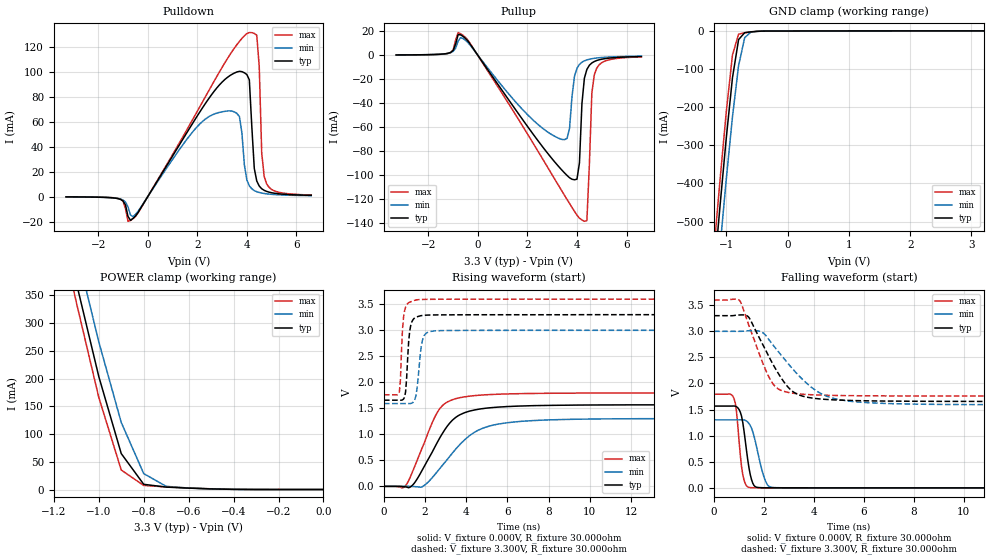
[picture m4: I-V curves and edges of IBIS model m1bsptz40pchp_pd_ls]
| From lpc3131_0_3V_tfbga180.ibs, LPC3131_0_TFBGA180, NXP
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| |   Rev 0.20 IBIS Model Design Automation Generation   |
| |   N O N - S I L I C O N   C O R R E L A T E D   |
| |   This IBIS [Model] is pre-Beta tactical support   |
| |  Note: this IBIS [Model] contains clamp curves generated   |
| |   through simulation which should not be relied upon   |
| Date/Time   : 2010 Jan 25 (Mon) 11:58:19
| Pccmos090 jliolib_p50 2.0
|   0.9 um 3.3V pad library
|   seven level metal
|   dual oxide
|   dual threshold voltage
|   nominal line mixed supply
|   parasitic extracted netlists
| Process block a10
| mem1bsptz40pchp
|   Bidirectional Pad 3.3
|   3state Output
|   Plain Input
|   CMOS
|   Programmable between
|   - (p1=0, p2=1) plain input
|   - (p1=0, p2=0) with Pull Up
|   - (p1=1, p2=1) with Pull Down
|   - (p1=1, p2=0) with Repeater
| Pull Down Mode low speed(esh=1, p1=1, p2=1)
[Model]   m1bsptz40pchp_pd_ls | of mem1bsptz40pchp
Model_type   I/O
Polarity   Non-Inverting
Enable   Active-Low
|  Reciever Thresholds
Vinl   = 0.99V
Vinh   = 2.31V
| AC Test Load Conditions
Vref   = 0
Cref   = 0
Rref   = 1000000000
Vmeas   = 1.65
| [Process Range]   typical   min   max
| C_comp edge width   400.000ps   400.000ps   400.000ps
| C_comp Tstrobe   40.000fs   40.000fs   40.000fs
C_comp   200.000pF   200.000pF   200.000pF
[Temperature Range]   25   125   -40
[Voltage Range]   3.30V   3.00V   3.60V
[GND Clamp Reference]   0.00V   0.00V   0.00V
[Pulldown Reference]   0.00V   0.00V   0.00V
[POWER Clamp Reference]   3.30V   3.00V   3.60V
[Pullup Reference]   3.30V   3.00V   3.60V
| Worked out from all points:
|   slope of the pulldown table from 0 to 0.495 V, typ, clamps not added: 30.9 ohm
|   slope of the pullup table from 0 to 0.495 V, typ, clamps not added: 33.2 ohm
|   GND clamp passes 1 mA (typ) near -0.51 V on its own axis
|   POWER clamp passes 1 mA (typ) near -0.45 V on its own axis
|   rising waveform, V_fixture 0.000V, R_fixture 30.000ohm: 20-80 % time 1.42ns typ, 1.87ns min, 1.15ns max; typ from 0 V to 1.57 V
|   falling waveform, V_fixture 0.000V, R_fixture 30.000ohm: 20-80 % time 277ps typ, 395ps min, 212ps max; typ from 1.57 V to 0 V
|   rising waveform, V_fixture 3.300V, R_fixture 30.000ohm: 20-80 % time 165ps typ, 222ps min, 139ps max; typ from 1.66 V to 3.3 V
|   falling waveform, V_fixture 3.300V, R_fixture 30.000ohm: 20-80 % time 1.16ns typ, 1.66ns min, 885ps max; typ from 3.3 V to 1.66 V
[GND Clamp]
| ref voltage   0.00V   0.00V   0.00V
|   Voltage   I(typ)   I(min)   I(max)
-3.3V     -4.732A    -4.814A    -4.684A
-1.2V     -636mA     -742.5mA   -569.7mA
-1.1V     -453.5mA   -561.8mA   -385.7mA
-1V       -279mA     -387.5mA   -210.8mA
-900mV    -122.8mA   -225.5mA   -63.13mA
-800mV    -22.45mA   -90.49mA   -8.204mA
-700mV    -4.394mA   -17.31mA   -4.534mA
-600mV    -2.163mA   -3.055mA   -2.529mA
-300mV    -78.17uA   -69.01uA   -98.11uA
3.2V      308.4uA    167.8uA    522.1uA
[Power Clamp]   | Vtable = Vcc - Vpad
| ref voltage   3.30V   3.00V   3.60V
|   Voltage   I(typ)   I(min)   I(max)
-3.3V     4.647A     4.675A     4.636A
-1.2V     553.3mA    610.4mA    520.8mA
-1.1V     373.2mA    433.6mA    337.9mA
-1V       204.1mA    266.6mA    166.5mA
-900mV    65.1mA     121.2mA    35.47mA
-800mV    9.693mA    28.95mA    7.599mA
-700mV    4.658mA    6.108mA    5.079mA
-600mV    2.822mA    2.869mA    3.125mA
-400mV    573.3uA    634.5uA    703uA
0V        308.5uA    161.6uA    522.8uA
[Pulldown]
| ref voltage   0.00V   0.00V   0.00V
|   Voltage   I(typ)   I(min)   I(max)
-3.3V     -236.7uA   -252.6uA   -192uA
-1.2V     -1.652mA   -1.556mA   -1.496mA
-600mV    -17.54mA   -16.01mA   -17.75mA
2.9V      89.5mA     67.39mA    99.97mA
3.7V      100.2mA    63.94mA    124.2mA
4.1V      93.4mA     8.546mA    131.2mA
4.3V      22.52mA    4.759mA    130.5mA
4.4V      12.45mA    3.873mA    129.1mA
4.5V      8.402mA    3.255mA    104mA
4.6V      6.246mA    2.801mA    34.93mA
4.8V      4.127mA    2.184mA    10.1mA
6.6V      979.6uA    712.7uA    1.221mA
[Pullup]   | Vtable = Vcc - Vpad
| ref voltage   3.30V   3.00V   3.60V
|   Voltage   I(typ)   I(min)   I(max)
-3.3V     207.2uA    209.5uA    174.1uA
-500mV    13.97mA    12.41mA    14.82mA
3.4V      -96.32mA   -70.52mA   -113.9mA
3.7V      -102.5mA   -61.11mA   -124.1mA
3.9V      -104.2mA   -17.59mA   -130.7mA
4.1V      -89.97mA   -7.665mA   -136.3mA
4.2V      -40.47mA   -5.865mA   -137.9mA
4.3V      -19.14mA   -4.724mA   -138.9mA
4.4V      -11.89mA   -3.942mA   -138.3mA
4.6V      -6.502mA   -2.948mA   -31.69mA
4.7V      -5.28mA    -2.614mA   -16.33mA
6.6V      -1.118mA   -810uA     -1.413mA
[Ramp]
R_load   = 30.000ohm
|   dV/dt(typ)   dV/dt(min)   dV/dt(max)
dV/dt_r   940.465mV/1.400ns   781.921mV/1.900ns   1.077V/1.150ns
dV/dt_f   985.822mV/1.150ns   844.534mV/1.700ns   1.103V/850.000ps
[Rising Waveform]  | cubic spline decimation from 501 points
V_fixture   = 0.000V
R_fixture   = 30.000ohm
|   Time   V(typ)   V(min)   V(max)
0s        3.993nV    181.6nV    2.818nV
950ps     -5.394mV   33.03uV    -20.12mV
1.35ns    8.653mV    -1.865mV   245.1mV
1.9ns     341.7mV    2.846mV    778.9mV
2.65ns    887.5mV    312mV      1.458V
3.2ns     1.218V     578.3mV    1.644V
3.7ns     1.378V     808.7mV    1.705V
4.95ns    1.502V     1.138V     1.76V
7.25ns    1.551V     1.264V     1.785V
25ns      1.567V     1.303V     1.795V
[Falling Waveform]  | cubic spline decimation from 501 points
V_fixture   = 0.000V
R_fixture   = 30.000ohm
|   Time   V(typ)   V(min)   V(max)
0s        1.567V     1.303V     1.795V
800ps     1.568V     1.303V     1.711V
900ps     1.554V     1.303V     1.451V
1.05ns    1.452V     1.304V     630.5mV
1.15ns    1.251V     1.304V     249mV
1.4ns     377.6mV    1.231V     8.832mV
1.65ns    22.24mV    894.1mV    1.709mV
2.05ns    1.746mV    141.1mV    782.3uV
2.35ns    933.5uV    7.946mV    592.2uV
25ns      16.41nV    230.3nV    23.85nV
[Rising Waveform]  | cubic spline decimation from 501 points
V_fixture   = 3.300V
V_fixture_min = 3.000V
V_fixture_max = 3.600V
R_fixture   = 30.000ohm
|   Time   V(typ)   V(min)   V(max)
0s        1.656V     1.591V     1.759V
750ps     1.655V     1.591V     1.818V
800ps     1.655V     1.591V     2.042V
900ps     1.662V     1.591V     3.011V
1ns       1.712V     1.591V     3.372V
1.25ns    2.977V     1.591V     3.54V
1.6ns     3.257V     1.86V      3.585V
1.9ns     3.286V     2.847V     3.592V
2.4ns     3.294V     2.985V     3.595V
25ns      3.299V     2.999V     3.598V
[Falling Waveform]  | cubic spline decimation from 501 points
V_fixture   = 3.300V
V_fixture_min = 3.000V
V_fixture_max = 3.600V
R_fixture   = 30.000ohm
|   Time   V(typ)   V(min)   V(max)
0s        3.299V     2.999V     3.598V
1ns       3.312V     2.999V     3.599V
1.35ns    3.287V     3.009V     3.173V
1.9ns     2.792V     2.987V     2.453V
2.3ns     2.42V      2.774V     2.034V
2.6ns     2.171V     2.594V     1.887V
3.15ns    1.847V     2.278V     1.814V
4.35ns    1.699V     1.79V      1.776V
5.95ns    1.669V     1.638V     1.764V
25ns      1.656V     1.591V     1.759V
